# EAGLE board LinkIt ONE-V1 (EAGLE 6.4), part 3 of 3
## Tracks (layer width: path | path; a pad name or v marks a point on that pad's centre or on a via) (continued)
SMPSLDO_1V6  (via drill 0.3 pad 0.51) (continued)
  GND 0.406: C19.2 58.85,80.9 58.85,81.76 | 54.67,79.56 53.91,79.56 | 53.91,79.56 52.92,79.56 v52.91,79.58 | v54.28,80.77 54.28,79.96 | 54.28,79.96 54.28,79.93 53.91,79.56 | 54.28,79.96 54.67,79.56 | 58.85,81.76 58.85,82.35 v58.83,82.37 | v59.11,81.76 58.85,81.76 | v57.81,79.2 C19.2 | 54.67,79.56 57.47,79.56 | 57.47,79.56 57.52,79.56 C19.2 | 57.47,79.56 57.79,79.25
  Bottom 0.152: 58.29,81.51 U1.D10 58.28,81.55 58.45,81.71 59.05,81.71 v59.11,81.76 | U1.C3 U1.C2 54.23,81.02 54.23,80.77 v54.28,80.77 | U1.E10 58.5,82.05 v58.83,82.37
  Bottom 0.203: U1.A8 57.26,79.9 57.81,79.35 v57.81,79.2
  Bottom 0.305: 54.23,80.77 54.23,81.09 54.67,81.09 54.74,81.03
  Bottom 0.406: v52.91,79.58 51.54,79.58 C11.1 50.42,76.66 L6.1
SPI_MISO  (via drill 0.3 pad 0.51)
  Top 0.152: 26.95,103.86 v26.95,103.81 28.63,105.49 30.3,105.49 U11.13 | v34.57,90.02 34.57,89.59 34.93,89.23 37.47,89.23 38.18,88.52 41.07,88.52 42.09,89.53 46.71,89.53 47.73,88.52 51.49,88.52 52.55,87.45 60.91,87.45 61.87,86.49 U11.38
  Bottom 0.152: v26.95,103.81 26.99,103.77 U18.13 26.99,101.58 27.36,101.22 27.36,100.81 24.72,98.18 24.72,92.24 27.98,88.98 31.98,88.98 32.79,89.79 33.25,89.79 33.4,89.64 34.19,89.64 v34.57,90.02
SPI_MOSI  (via drill 0.3 pad 0.51)
  Top 0.152: U11.34 65.51,83.95 64.24,85.22 62.61,85.22 60.68,87.15 52.45,87.15 51.38,88.21 47.62,88.21 46.61,89.23 42.19,89.23 41.17,88.21 38.02,88.21 37.31,88.92 34.77,88.92 v33.58,90.12 | U11.12 32.54,105.18 28.98,105.18 v27.61,103.81
  Bottom 0.152: v27.61,103.81 27.61,102.49 27.66,102.44 27.66,102.25 U18.14 27.64,100.59 25.01,97.96 25.01,92.39 28.12,89.28 31.67,89.28 32.51,90.12 v33.58,90.12
SPI_SCL  (via drill 0.3 pad 0.51)
  Top 0.152: U11.37 63.37,83.95 60.48,86.84 52.35,86.84 51.28,87.91 47.52,87.91 46.51,88.92 42.29,88.92 41.28,87.91 37.82,87.91 37.11,88.62 34.47,88.62 33.71,89.38 33.07,89.38 v33,89.31 | U11.14 29.08,106.66 v26.24,103.81
  Bottom 0.152: v26.24,103.81 26.34,103.71 U18.12 | U18.12 | v33,89.31 32.36,88.67 27.86,88.67 24.4,92.14 24.4,98.36 26.29,100.25 26.29,100.46 26.29,102.17 U18.12
SPI_SS  (via drill 0.3 pad 0.51)
  Top 0.152: U11.11 35.94,106.81 34.01,104.88 29.34,104.88 v28.27,103.81
  Bottom 0.152: v28.27,103.81 U18.15
SQI_CE  (via drill 0.1 pad 0.25 layers 15-16, 0.2 pad 0.41 layers 2-15, 0.3 pad 0.51)
  GND 0.152: v36.26,79.43 36.92,79.43 37.24,79.75 37.24,80.16 36.91,80.49 36.91,86.69 v36.65,86.94
  GND1 0.076: v36.26,79.43 36.26,79.36 v36.07,79.16
  Bottom 0.102: 38.54,85.78 U3.1
  Bottom 0.152: v36.65,86.94 38.12,86.94 38.53,86.54 38.53,85.78 U3.1 | U7.G13 36.14,79.09 v36.07,79.16
SQI_SCK  (via drill 0.1 pad 0.25 layers 15-16)
  GND1 0.076: U7.G8 36.41,77 36.41,77.28 36.26,77.43 36.26,77.62 36.1,77.78 36.1,78.57 37.21,79.68 37.21,80.49 36.65,81.05 v36.65,81.15
  Bottom 0.102: U3.6 32.05,83.21 31.93,83.08 31.93,81.41 32.08,81.25 36.55,81.25 v36.65,81.15
  other vias: 36.14,76.73
SQI_SI  (via drill 0.1 pad 0.25 layers 15-16)
  GND1 0.076: v36.96,77.5 36.92,77.54 36.92,78.15 37.56,78.8 37.56,80.91 37.56,81.05 v37.16,81.46
  Bottom 0.076: U7.F9 36.59,77.13 v36.96,77.5
  Bottom 0.102: U3.5 32.81,81.6 32.95,81.46 v37.16,81.46
SQI_SIO2
  Bottom 0.076: U7.F12 36.54,78.43 36.54,78.45 36.54,79.43 36.86,79.75
  Bottom 0.102: 38.59,83.19 U3.3 38.59,83.24 39.35,83.24 39.6,82.98 39.6,81.66 39.59,81.66 39.29,81.36 38.46,81.36 36.86,79.75
SQI_SIO3  (via drill 0.1 pad 0.25 layers 15-16)
  GND1 0.076: v37.11,81.05 37.38,80.78 37.38,78.84 36.76,78.22 36.76,77.74 U7.F10
  Bottom 0.102: U3.7 31.95,84.48 31.67,84.2 31.67,81.3 31.93,81.05 36.3,81.05 36.55,80.8 36.86,80.8 v37.11,81.05
  other vias: 36.54,77.53
SQI_SO
  Bottom 0.076: 36.78,79.95 36.39,79.56 36.39,78.56 36.15,78.33 U7.G12
  Bottom 0.102: 38.54,84.51 U3.2 37.85,84.48 37.67,84.3 37.67,80.84 36.78,79.95
SW_SPI/SDIO  (via drill 0.3 pad 0.51)
  Top 0.152: U6.10 31.45,91.95 31.52,92.02 31.55,92.05 31.55,93.47 v31.52,93.5 | U6.2 26.59,92.45 v26.39,92.25 | v31.52,93.5 v31.52,93.49 v31.52,93.5 | SW1.COM 28.02,83.44 v27.46,84
  GND 0.152: v31.52,93.5 31.11,93.09 27.25,93.09 26.41,92.25 v26.39,92.25 25.02,90.88 v25.02,90.04
  Bottom 0.152: v25.02,90.04 26.92,88.14 26.92,86.61 27.56,85.98 27.56,84.1 v27.46,84
TR_N
  Bottom 0.114: L7.1 63.95,78.36 64.35,78.36 C141.1 64.59,78.54 64.77,78.36 65.05,78.36 arc45 65.22,78.43 65.53,78.74 65.86,78.74 U15.7
TR_P
  Bottom 0.076: 63.94,77.96 63.92,77.96 R61.1 | 64.85,77.95 64.83,77.95 C141.2
  Bottom 0.114: U15.5 65.56,77.51 65.19,77.88 arc45 65.01,77.95 64.85,77.95 | 63.94,77.96 64.35,77.96 C141.2
TRX_IO_N
  Bottom 0.114: U1.C10 58.3,81.05 58.31,81.04 arc45 58.52,80.96 58.58,80.96 arc-45 58.85,80.84 61.23,78.47 arc90 61.77,78.47 C142.1 61.9,78.56 62.1,78.36 62.55,78.36 L7.2
TRX_IO_P
  Bottom 0.114: U1.B10 58.3,80.55 arc-45 58.53,80.64 58.45,80.64 arc-45 58.72,80.53 61.14,78.11 arc45 61.41,78 61.46,78 arc-45 61.73,77.88 C142.2 62.13,77.94 62.13,77.96 62.58,77.96 62.58,77.94 R61.2
TX_EN  (via drill 0.1 pad 0.25 layers 1-2, 0.1 pad 0.25 layers 15-16, 0.2 pad 0.41 layers 2-15, 0.3 pad 0.51)
  Top 0.152: v45.44,80.24 45.44,74.78 46.97,73.25 46.97,66.85 50.55,63.27 v50.72,63.27
  GND 0.152: v45.44,80.24 44.83,80.24 44.02,81.05 v43.92,81.05
  GND1 0.102: v40.09,76.91 40.09,77.22 40.72,77.85 40.72,80.07 42.05,81.41 43.56,81.41 v43.92,81.05
  Bottom 0.076: U7.A9 38.54,77.15
  Bottom 0.102: U7.A9 39.88,77.13 v40.09,76.91
  Bottom 0.152: R55.2 R75.2 51.4,64.1 50.72,63.42 v50.72,63.27
TXO_HB
  Bottom 0.102: U7.C2 37.67,74.24 37.67,73.33
  Bottom 0.132: 37.67,73.33 37.67,70.43 arc45 37.78,70.16 40.9,67.04 arc45 41.17,66.93 48.32,66.93 arc45 48.7,67.08 49.01,67.4 arc-45 49.47,67.59 C134.1 L16.2
TXO_LB
  Bottom 0.102: U7.B2 38.14,74.31 37.93,74.09 arc45 37.87,73.97 37.87,73.62 arc45 37.93,73.47 37.97,73.43
  Bottom 0.132: 37.97,73.43 38.21,73.2 arc-45 38.33,72.91 38.33,70.7 arc45 38.44,70.43 41.24,67.63 arc45 41.51,67.52 47.94,67.52 arc45 48.14,67.6 49.24,68.69 arc-45 49.52,68.81 C135.1 L1.2
UART1_RX  (via drill 0.1 pad 0.25 layers 15-16, 0.2 pad 0.41 layers 2-15, 0.3 pad 0.51)
  Top 0.152: 30.87,102.44 R106.2 31.43,102.43 31.72,102.13 31.72,100.51 v31.77,100.46
  GND 0.152: v40.82,81.41 40.64,81.58 40.64,87.07 42.64,89.08 43.94,89.08 45.24,90.38 45.24,92.23 35.74,101.73 v35.74,101.85
  GND1 0.076: v37.18,77.18 37.34,77.18 37.44,77.28 38.08,77.28 38.15,77.21 38.61,77.21 38.93,77.53 39.33,77.53 39.98,78.19 39.98,78.79 39.63,79.14 39.63,80.06 39.74,80.18 39.74,81.04 40.11,81.41 v40.82,81.41
  Bottom 0.076: U7.E9 37.12,77.13 v37.18,77.18
  Bottom 0.152: v31.77,100.46 32.07,100.46 32.7,101.09 34.4,101.09 R82.2 35.34,101.85 v35.74,101.85 36.12,101.85 Q9.2 36.25,101.73
UART1_TX  (via drill 0.1 pad 0.25 layers 15-16, 0.2 pad 0.41 layers 2-15, 0.3 pad 0.51)
  Top 0.152: 27.5,102.43 26.8,101.73 v26.8,101.07
  Top 0.203: R107.2 27.5,102.43
  GND 0.152: v40.97,80.9 41.22,81.15 41.22,81.66 40.92,81.97 40.92,86.79 42.85,88.72 44.02,88.72 45.54,90.25 45.54,92.38 39.09,98.83 v39.09,99.75 | v26.8,101.07 30.5,101.07 33,98.58 35.18,98.58 v35.74,98.02
  GND1 0.076: U7.E8 37.13,76.73 37.53,77.12 38.01,77.12 38.09,77.05 38.8,77.05 38.96,76.89 39.24,76.89 40.34,77.98 40.34,79.5 39.9,79.93 39.9,80.7 40.11,80.9 v40.97,80.9
  GND1 0.102: 41.06,80.98 v40.97,80.9
  Bottom 0.152: v35.74,98.02 36.37,98.02 Q8.2 36.45,98.22 37.31,99.09 39.21,99.09 R46.2 39.46,99.38 v39.09,99.75
  other vias: 36.94,76.73
USB_5V  (via drill 0.3 pad 0.51, 0.38 pad 0.64)
  Top 0.152: R33.1 15.54,73.34 15.54,75.18 15.93,75.57 U12.2
  Top 0.406: 4.96,84.2 5.1,84.35 | U12.2 17.52,75.57 17.78,75.31 17.78,74.08 | 8,78.23 8,78.68 C49.+ | C106.1 17.82,73.7 v18.41,74.3
  Top 1.016: 5.1,84.35 5.18,84.35 v5.66,84.84
  GND 0.61: v7.75,77.34 5.84,77.34 3.05,74.55 3.05,65.53 v5.21,63.37 6.12,62.46 v6.12,58.74
  GND 2.032: 7.62,77.34 v7.75,77.34 8.64,77.34 9.91,77.34 10.03,77.34 10.67,76.71 11.05,76.33 13.08,74.3 v18.41,74.3
  Bottom 0.152: v18.41,74.3 18.41,74.4 18.92,74.91
  Bottom 0.203: R70.1 8.37,59.36 13.01,59.36 VCHG_5V1.T | 18.92,74.93 19.24,74.93 C74.1
  Bottom 0.406: 6.13,58.73 v6.12,58.74 | U8.4 4.83,58.74
  Bottom 0.61: 4.32,59.18 4.76,58.74 4.83,58.74 v6.12,58.74 C116.1 R70.1 | 4.19,63.25 Q14.2 v5.21,63.37 6.29,63.37 R93.1
  Bottom 1.778: v5.66,84.84 5.66,79.43 v7.75,77.34
  other vias: 18.03,74.93 19.05,74.17 6.98,77.34 7.37,77.98
  pour Top (isolate 0.254, no thermals): 3.63,84.81 5.26,84.81 5.26,83.85 3.63,83.85
  pour Bottom (isolate 0.254, no thermals): 17.53,75.56 17.53,74.3 arc90 17.78,74.04 19.56,74.04 arc90 19.81,74.3 19.81,75.56 arc90 19.56,75.82 17.78,75.82 arc90
  pour Top (isolate 0.254, no thermals): 17.53,74.42 17.4,74.42 arc90 17.14,74.17 17.14,73.71 arc90 17.4,73.46 19.05,73.46 arc90 19.3,73.71 19.3,75.18 arc90 19.05,75.44 17.78,75.44 17.78,74.68 arc-90
  pour Top (isolate 0.254, no thermals): 6.6,78.26 7.24,78.26 arc90 7.49,78.51 7.49,79.88 arc-90 7.75,80.14 8.64,80.14 arc-90 8.89,79.88 8.89,77.22 arc-90 8.64,76.96 6.6,76.96 arc-90 6.35,77.22 6.35,78 arc-90
USB_N
  Top 0.114: J7.2 5.53,83.33 5.71,83.14 6.59,83.14 | 6.59,83.14 7.56,83.14 R17.1 | 6.59,83.14 6.59,83.93 DP.T
USB_P
  Top 0.114: J7.3 5.57,82.68 5.71,82.82 6.6,82.82 | 6.6,82.82 7.69,82.82 R18.1 | 6.6,82.82 DN.T
USBD_N  (via drill 0.3 pad 0.51)
  Top 0.114: R17.2 9.02,83.64 9.47,83.19 10.09,83.19 10.24,83.34 D6.1 12.81,83.92 13.54,83.19 21.27,83.19 25.95,78.52 31.84,78.52 32.23,78.13 v32.23,77.9
  Bottom 0.076: U7.N11 33.49,77.68 32.46,77.68 v32.23,77.9
  Bottom 0.102: U7.N11 33.7,77.93
USBD_P  (via drill 0.3 pad 0.51)
  Top 0.114: R18.2 9.05,82.45 9.47,82.87 10.09,82.87 10.24,82.73 D6.2 12.81,82.14 13.54,82.87 21.14,82.87 25.82,78.2 31.52,78.2 v31.62,78.1
  Bottom 0.076: U7.P11 32.92,77.93 32.51,78.34 31.86,78.34 v31.62,78.1
VA  (via drill 0.1 pad 0.25 layers 1-2, 0.1 pad 0.25 layers 15-16, 0.2 pad 0.41 layers 2-15)
  Top 0.152: v31.93,74.3 32.12,74.3 C94.1
  GND 0.132: v32.33,74.3 v31.93,74.3 v32.33,74.3
  GND1 0.132: v32.74,74.4 32.64,74.3 v32.33,74.3
  Bottom 0.152: 33.33,74.73 U7.P3 33.27,74.73 32.94,74.4 v32.74,74.4
VBAT  (via drill 0.1 pad 0.25 layers 1-2, 0.1 pad 0.25 layers 15-16, 0.2 pad 0.41 layers 2-15, 0.3 pad 0.51)
  Top 0.152: 37.3,73.1 37.14,73.1 v36.78,73.46 | 41.1,65.58 41.1,65.63 v41.17,65.71
  Top 0.203: 34.8,76.36 C72.1 | 36.07,62.36 37.52,62.36 v37.67,62.2 | v34.72,74.7 34.72,74.77 C101.1
  Top 0.254: U20.6 21.9,67.11 21.34,66.55 19.56,66.55 18.99,67.11 U20.3
  Top 0.305: C33.+ 40.44,62.74 40.46,62.76 40.46,62.92 | 37.33,73.18 C8.1 | R78.2 12.76,58.86 13.46,59.56 15.88,59.56 v16.13,59.31
  Top 0.406: v33.96,76.38 C72.1 | C3.1 30.73,66.8 30.17,66.24
  Top 0.61: U4.1 52.77,91.12 C45.1 52.4,91.06 v51.41,90.07 | 37.59,71.88 C73.1 | C73.1 37.35,72.12 C8.1 37.3,73.1 37.28,73.1 35.33,75.06 35.07,75.06 C101.1 35.03,75.82 34.81,76.03 C72.1 34.82,76.36 | 38.25,66.02 38.25,65.81 37.85,65.41 | 38.25,66.02 38.25,66.06 | 38.25,66.06 38.25,71.22 C73.1 | v51.13,66.67 50.42,67.39 50.42,77.52 | 50.42,77.52 50.42,77.6 48.64,79.38 48.64,81.47 v48.88,81.71 | 50.42,77.52 L2.1 | 38.25,66.02 38.86,65.41 | 38.25,66.06 37.72,65.53
  Top 1.016: C50.+ 30.8,65.62 30.79,65.63 | v41.17,65.71 40.87,65.41 38.86,65.41 37.85,65.41 v36.65,65.41 v35.89,65.41
  Top 1.27: v35.89,65.41 35.64,65.41 v35.13,65.91
  Top 2.032: C30.+ C33.+ | 35.94,62.48 36.07,62.36 36.07,62.51 C30.+ | C30.+ 35.89,62.69 v35.89,65.41 35.71,65.58 30.84,65.58 30.79,65.63 30.17,66.24 28.3,68.12 27.06,68.12 L8.1
  GND 0.152: v60.43,63.93 60.43,64.59 61.09,64.59 v61.14,64.64 60.45,64.64 | 60.43,65.15 v60.38,65.2 | v37.67,62.2 37.67,62.31 v38.18,62.81 38.23,62.76 38.23,62.74 | v38.63,62.23 38.63,62.33 38.23,62.74 | 38.23,62.74 38.23,62.36 | v34.27,74.45 34.47,74.45 v34.72,74.7 | v33.93,70.08 33.48,69.62 33.15,69.62 32.74,70.03 29.29,70.03 28.42,70.89 13.39,70.89 11.1,73.18 6.43,73.18 6.22,72.97 SW3.COM2 | v36.6,73.74 36.6,73.63 v36.78,73.46
  GND 0.203: v33.96,76.38 33.96,76.76 33.81,76.91 v33.81,77.57
  GND 0.305: 17.53,69.22 17.53,69.62 | v15.24,68.77 15.24,69.49 | 15.24,69.49 15.37,69.62 | 15.24,69.49 15.24,69.8 15.27,69.83
  GND 0.61: v41.17,65.71 50.16,65.71 v51.13,66.67 | v51.41,90.07 50.01,88.67 50.01,82.84 v48.88,81.71
  GND 2.032: 60.45,64.64 57.79,64.64 54.17,61.02 39.56,61.02 38.23,62.36 | SW3.COM1 SW3.COM2 10.57,71.88 12.83,69.62 15.37,69.62 17.53,69.62 27.84,69.62 32.05,65.41 v35.89,65.41
  GND1 0.102: U7.M10
  GND1 0.132: U7.E1 36.75,73.74 v36.6,73.74
  GND1 0.152: U7.L3 v34.27,74.45 | v33.81,77.57 34.1,77.57 U7.M10
  Bottom 0.102: U7.H1 35.74,73.89 35.64,73.79 35.64,73.18 34.21,71.75 34.21,71.14 33.93,70.87 v33.93,70.08
  Bottom 0.152: C128.2 60.38,64.64 | 60.38,64.64 60.43,64.59 | 60.38,64.64 v61.14,64.64
  Bottom 0.305: U14.26 56.56,65.26 56.77,65.05 | v16.13,59.31 15.68,59.76 15.68,63.88 | 15.68,63.88 15.68,66.23 15.88,66.42 15.88,66.41 D2.2 15.89,68.12 15.83,68.18 v15.24,68.77 | 15.68,63.88 15.43,63.63 VBAT_TP.T 15.37,63.63 15.62,63.37
  other vias: 34.54,74.73 34.14,77.53 36.94,73.93
  pour Bottom (isolate 0.254, no thermals): 56.46,66.42 56.67,66.42 56.67,65.76 56.93,65.51 60.86,65.51 arc-90 61.49,64.87 61.49,64.36 arc-90 60.86,63.73 58.62,63.73 arc-90 58.24,64.11 arc90 57.61,64.74 56.46,64.74
  pour Top (isolate 0.254, no thermals): 22.22,67.31 23.57,67.31 23.75,67.49 23.75,68.83 arc-90 24.38,69.47 28.45,69.47 arc-90 29.08,68.83 29.08,67.49 arc-90 28.45,66.98 22.22,66.98
VCDT  (via drill 0.1 pad 0.25 layers 15-16, 0.3 pad 0.51)
  GND 0.152: v31.22,69.42 31.22,68.61 32.33,67.49 v32.33,67.13 | v8.28,57.84 8.28,61.48 9.16,62.36 9.91,62.36 10.41,61.85 16.76,61.85 v17.27,62.36
  GND1 0.102: v35.33,75.13 35.33,73.83 34.12,72.62 33.35,72.62 33.2,72.47 33.2,72.11 v33.15,72.06
  Bottom 0.102: 35.35,75.13 U7.J4 v35.33,75.13
  Bottom 0.152: v33.15,72.06 33.15,71.68 31.22,69.75 v31.22,69.42 | v32.33,67.13 23.24,67.13 18.72,62.61 17.53,62.61 v17.27,62.36 | R86.1 8.78,57.84 v8.28,57.84 7.76,57.84 R70.2
VCORE  (via drill 0.1 pad 0.25 layers 15-16, 0.3 pad 0.51)
  Top 0.406: 38.23,78.1 38.28,78.16 | 38.23,78.1 38.28,78.1 | 38.28,78.1 37.67,77.5 33.26,77.5 v32.88,77.12 | 38.28,78.1 39.02,78.1 v39.07,78.05 | 38.23,78.1 38.23,78.12 C69.1
  GND1 0.076: v32.88,77.12 U7.P9
  Bottom 0.152: U7.A11 38.94,77.93 v39.07,78.05
  other vias: 33.34,77.13
VIO18_LDO  (via drill 0.3 pad 0.51)
  Top 0.406: v32.94,79.78 33.15,79.78 33.41,80.05 R37.1 C70.1 32.27,80.91 31.77,81.41 30.96,81.41 v30.61,81.05
  Bottom 0.152: U7.P13 U7.N13 33.74,79.19 33.15,79.78 v32.94,79.78
  Bottom 0.406: 30.77,86.31 31.56,87.1 34.87,87.1 35.94,88.16 39.35,88.16 39.84,87.66 40.59,87.66 41.09,88.16 R114.1 | 30.77,86.31 30.71,86.24 | 30.77,86.31 30.77,86.3 30.56,86.08 30.56,81.1 v30.61,81.05 | 41.68,89.53 41.5,89.71 41.5,89.76 Q11.1 | 41.07,93.13 R118.1 41.58,93.14 | 41.78,92.96 41.78,90.04 Q11.1 | 41.78,92.96 41.78,93.34 | 41.78,93.34 41.78,94.28 Q13.1 41.55,94.51 42.17,95.13 42.17,99.21 41.99,99.39 41.54,99.39 R115.1 41.5,101.5 Q12.1 | 41.58,93.14 41.78,93.34 | 41.58,93.14 41.61,93.14 41.78,92.96 | Q11.1 41.09,89.34 R114.1 | 41.15,88.38 41.11,88.38 R114.1
VIO28_LDO  (via drill 0.3 pad 0.51)
  Top 0.152: v52.91,83.21 52.98,83.21 54.08,84.3 54.97,84.3 55.27,84.61 56.17,84.61 C23.1
  Top 0.203: R53.2 v6.98,107.06 | v39.29,76.35 40.14,76.35 40.16,76.38
  Top 0.406: C71.1 C63.1 38.34,76.35 v39.29,76.35 40,76.35 R67.1 40.16,76.38 40.77,76.38 41.22,76.83 42.55,76.83 | C23.1 56.74,85.2 v56.74,86.23 56.74,86.34 arc-45 56.77,86.4 | 58.19,86.4 60.12,86.4 60.59,85.92 R92.2 R87.2 | v58.45,85.52 58.45,86.13 | v42.55,87.71 42.7,87.86 46.17,87.86 47.19,86.84 51.61,86.84 52.06,86.4 56.77,86.4 | v45.97,81.74 45.87,81.74 44.76,80.62 44.21,80.62 42.8,79.21 42.8,77.09 | 42.8,76.58 42.8,73.86 43.21,73.46 v43.21,63.09 43.21,60.88 44.27,59.82 46.97,59.82 47.62,59.16 v47.62,58.8 | 42.8,76.58 42.8,77.09 | 42.55,76.83 42.8,77.09 | 42.55,76.83 42.8,76.58 | 56.77,86.4 58.19,86.4 | 58.19,86.4 58.45,86.14 58.45,86.13 | 58.45,86.13 58.65,86.33 | R76.2 29.16,102.56 28.52,103.2 26.39,103.2 | 26.39,103.2 25.98,103.2 | 26.19,103 25.98,103.2 | R77.2 26.19,103 | 26.19,103 26.39,103.2 | 19.84,103.2 v19.79,103.15 20.27,103.63 22.45,103.63 | v42.95,95.83 41.02,95.83 39.29,97.56 v38.23,97.56 | v38.12,92.63 41.71,92.63 v42.52,93.45 | 25.98,103.2 25.96,103.2 25.53,103.63 22.99,103.63 | 22.99,103.63 22.45,103.63 | R49.2 22.73,103.35 | 22.73,103.35 22.73,103.38 22.99,103.63 | 22.73,103.35 22.45,103.63
  Top 0.61: C14.2 54.83,80.3 v55.27,80.75
  GND 0.305: v30.86,95.07 | v30.86,95.07 28.99,95.07 26.8,97.26 23.44,97.26 21.31,95.12 v20.5,95.12 19.79,95.83 v19.79,103.15 | v6.98,107.06 7.34,107.06 10.03,104.37 18.57,104.37 v19.79,103.15 | 19.79,102.74 v19.79,103.15 | v30.86,95.07
  GND 0.406: 55.25,80.7 55.27,80.72 v55.27,80.75 55.9,80.12 57.21,80.12 58.15,81.06 58.15,84.51 58.45,84.81 v58.45,85.52 | v47.62,58.8 47.62,57.53 46.97,56.87 25.07,56.87 22.11,59.83 22.05,59.89 v22.05,60.76 | v33.1,92.43 33.15,92.43 33.25,92.53 33.25,93.43 32.04,94.64 31.29,94.64 v30.86,95.07
  Bottom 0.102: U7.B7 38.14,76.34 38.12,76.33
  Bottom 0.152: U1.H1 53.48,83.55 53.15,83.21 v52.91,83.21 | U1.D3 55.27,81.03 v55.27,80.75 | U17.6 45.66,62.49 45.44,62.71 45.44,63.47 45.14,63.78 44.56,63.78 U17.3 | 21.25,60.5 R36.2 | VIO_28.T 16.73,63.08 16.73,61.63 17.14,61.21 19.54,61.21 R81.2
  Bottom 0.203: U1.J7 U1.K7 56.76,86.22 v56.74,86.23 | 38.12,76.33 38.12,76.71 U7.B8 | 38.14,76.34 39.28,76.34 v39.29,76.35
  Bottom 0.254: v58.45,85.52 58.45,84.91 58.26,84.72 U1.K10
  Bottom 0.305: U17.3 43.07,63.79 C122.1 42.98,63.7 | 20.26,60.5 R81.2 R36.2 21.81,60.52 v22.05,60.76
  Bottom 0.406: R69.1 C5.1 32.32,98.36 30.88,96.91 U18.2 30.88,95.08 v30.86,95.07 | Q3.1 31.48,92.48 R98.1 32.22,92.43 v33.1,92.43 33.86,92.43 34.9,91.39 Q4.1 36.34,91.39 R99.1 | C122.1 43.21,63.52 v43.21,63.09 | v45.97,81.74 45.97,83.19 42.55,86.61 v42.55,87.71 42.55,93.42 v42.52,93.45 42.52,94.18 42.95,94.61 v42.95,95.83 | v20.5,95.12 20.43,95.19 20.02,95.19 R38.1 | 36.39,91.44 R99.1 | 37.34,93.08 37.34,93.65 Q10.1 | 37.34,92.46 37.95,92.46 v38.12,92.63 | 37.34,92.46 36.77,92.46 36.51,92.19 R99.1 | R82.1 35.27,102.84 35.43,102.84 35.74,102.54 37.21,102.54 Q9.1 38.23,101.27 39.09,100.41 39.8,100.41 40.16,100.05 40.16,98.96 39.69,98.49 R46.1 38.6,98.49 38.08,97.97 38.1,97.97 Q8.1 v38.23,97.56 | 37.34,92.46 37.34,93.08 | 37.34,93.08 R112.1
VIO33_LDO  (via drill 0.3 pad 0.51)
  Top 0.305: U6.14 29.59,94.78 C87.1
  Top 0.406: 31.5,94.41 31.5,98.88 31.19,99.19 30.32,99.19 29.98,99.53 29.98,103 30.4,103.43 v30.86,103.43 30.86,103.4 | v35.08,94.06 35.08,94.11 34.22,93.25 32.65,93.25 31.5,94.41 | 31.5,94.41 30.86,94.41 | 30.86,94.41 30.61,94.41 30.05,94.97 C87.1 | v30.86,94.03 30.86,94.41
  GND 0.406: v41.94,102.79 41.89,102.79 40.21,104.47 31.32,104.47 30.86,104.01 v30.86,103.43 | v29.74,85.57 29.74,88.47 30.61,89.33 30.61,90.75 32.59,92.74 32.59,93.29 31.78,94.1 30.93,94.1 | 30.93,94.1 v30.86,94.03 30.93,94.1
  GND 0.61: v11.46,88.92 13.71,86.67 19.03,86.67 19.99,87.63 19.99,89.53 24.11,93.65 30.48,93.65 v30.86,94.03 | v31.37,63.88 31.24,63.88 27.05,68.07 12.07,68.07 v10.92,69.22
  Bottom 0.152: 31.95,94.28 32.02,94.28 R73.2 | R83.2 35.26,98.6
  Bottom 0.203: 30.86,102.24 U18.19
  Bottom 0.406: v30.86,103.43 30.88,103.41 U18.19 30.88,101.34 31.11,101.1 32.1,101.1 C7.1 34.04,102.02 R111.2 | 35.26,98.6 35.05,98.6 34.32,97.87 34.32,95.38 34.63,95.06 R113.2 35.1,94.08 v35.08,94.06 | R117.2 R119.2 44.86,102.09 R116.2 42.61,102.12 v41.94,102.79 | R20.1 29.55,85.33 29.74,85.52 v29.74,85.57 | v30.86,94.03 30.04,94.03 R71.2 | v30.86,94.03 30.86,94.06 | 32.04,94.21 R73.2 31.97,94.13 31.01,94.13 30.91,94.03 v30.86,94.03
  Bottom 0.61: v11.46,88.92 11.46,87.1 10.25,85.89 10.25,85 11.81,83.44 11.81,70.1 v10.92,69.22 | R116.2 45.11,101.89 C2.1 45.11,98.53 C32.1 45.14,96.44 U19.4 | v31.37,63.88 31.37,59.31 U11.31 30.61,58.42 32.13,56.9 34.04,56.9 U11.29
  pour Bottom (isolate 0.254, no thermals): 47.73,97.41 44.32,97.41 arc90 43.69,96.65 43.69,94.41 arc90 44.32,93.78 47.73,93.78 arc90 48.36,94.41 48.36,96.65 arc90
VMC  (via drill 0.1 pad 0.25 layers 15-16, 0.3 pad 0.51)
  Top 0.305: v24.75,77.99 25.96,76.78 30.64,76.78 31.2,76.22 C95.1 31.2,76.16 31.65,76.61 31.65,76.76 v31.67,76.78
  GND1 0.076: 32.81,76.73 32.95,76.73 33.36,76.33 33.55,76.33 33.98,76.76 34.57,76.76 U7.K9
  GND1 0.102: v31.67,76.78 31.78,76.67 32.58,76.67 32.64,76.73 32.81,76.73
  Bottom 0.305: 19.16,86.75 19.21,86.8 J4.4 19.85,86.8 20.55,87.5 R72.1
  Bottom 0.406: R2.1 R74.1 22.17,83.48 22.17,82.93 21.78,82.54 21.78,81.39 | 19.16,86.75 18.47,86.05 18.47,81.48 18.82,81.13 21.49,81.13 | 21.49,81.13 21.51,81.13 21.78,81.39 | v24.75,77.99 23.96,77.99 21.78,80.17 21.78,81.39 | 21.49,81.13 21.72,80.9 | C66.1 21.46,86.63 21.46,87.49 R72.1
  other vias: 34.94,77.13
VREF
  Bottom 0.152: U7.G1 36.14,73.31 34.7,71.87 C92.1
VRTC  (via drill 0.1 pad 0.25 layers 1-2, 0.1 pad 0.25 layers 15-16, 0.2 pad 0.41 layers 2-15)
  Top 0.406: D1.+ 18.29,86.54 18.29,85.34 19.3,84.33 21.46,84.33 | 21.84,84.33 21.46,84.33 | R8.1 21.65,84.52 | 21.65,84.52 21.46,84.33 | 21.65,84.52 21.84,84.33 | v30.4,79.58 30.35,79.63 26.92,79.63 26.54,80.01 26.54,80.97 25.97,81.53 24.89,81.53 22.1,84.33 21.84,84.33
  GND 0.203: v30.4,79.58 31.32,79.58 32.79,78.1 32.79,77.75 32.36,77.32 v32.3,77.32
  GND1 0.102: v32.3,76.99 v32.3,77.32
  Bottom 0.102: U7.P8 32.56,76.73 v32.3,76.99
VSF  (via drill 0.1 pad 0.25 layers 1-2, 0.1 pad 0.25 layers 15-16, 0.2 pad 0.41 layers 2-15, 0.3 pad 0.51)
  Top 0.152: v36.84,78.14 36.83,78.13
  Top 0.406: C47.1 v36.84,78.14
  GND 0.406: v36.2,87.5 36.25,87.55 36.96,87.55 37.31,87.2 37.31,80.7 37.64,80.37 37.64,79.61 v36.95,78.92 36.84,78.82 v36.84,78.14
  GND1 0.305: v36.38,78.02 36.38,78.35 v36.95,78.92
  Bottom 0.076: U7.F11 36.48,77.93 v36.38,78.02
  Bottom 0.406: U3.8 31.42,85.75 | 31.42,85.75 31.25,85.75 C91.1 | v36.2,87.5 35.21,86.52 31.81,86.52 31.42,86.13 31.42,85.75
VSIM1  (via drill 0.1 pad 0.25 layers 1-2, 0.1 pad 0.25 layers 15-16, 0.2 pad 0.41 layers 2-15, 0.3 pad 0.51)
  Top 0.152: v32.64,75.21 32.39,74.95 | C97.1 31.2,74.74
  Top 0.305: v30.96,74.93 31.01,74.93 31.2,74.74 32.17,74.74 v32.64,75.21
  GND 0.102: v33,75.41 32.79,75.21 v32.64,75.21
  GND 0.152: v5.1,94.28 5.1,94.26 5.77,93.6 8.76,93.6 v8.92,93.75 9.27,93.4 9.27,88.11 12.83,84.56 23.39,84.56 24.51,83.44 27.36,83.44 27.96,82.83 27.96,77.44 30.45,74.95 30.96,74.95 v30.96,74.93
  GND1 0.076: U7.L7 34.54,75.94 34.21,75.62 33.2,75.62 v33,75.41
  GND1 0.102: U7.L7 34.54,76.41
  Bottom 0.152: J4.C1 5.13,97.04 C65.1
  Bottom 0.203: J4.C1 5.13,94.31 v5.1,94.28 | J4.C6 8.94,93.77 v8.92,93.75
  other vias: 34.54,76.33
VSIM2  (via drill 0.3 pad 0.51)
  Top 0.152: C9.1 v36.2,79.98
  Bottom 0.076: v36.2,79.98 35.94,79.73 35.94,79.48 35.74,79.28 U7.H13
VUSB  (via drill 0.3 pad 0.51)
  Top 0.152: C10.1 32.27,79.41 32.54,79.15 32.92,79.15 v32.94,79.12
  Bottom 0.076: U7.P12 33.23,78.33
  Bottom 0.152: v32.94,79.12 32.94,78.61 33.23,78.33
WIFI_BT_PRI  (via drill 0.1 pad 0.25 layers 1-2, 0.1 pad 0.25 layers 15-16, 0.2 pad 0.41 layers 2-15, 0.3 pad 0.51)
  Top 0.152: R5.1 56.22,84.3 55.45,84.3 55.13,83.98 54.34,83.98 52.07,81.71 50.65,81.71 50.14,82.22 45.75,82.22 44.58,81.05 41.68,81.05 40.73,80.1 39.89,80.1 v39.8,80.19
  Top 0.406: R5.1 56.78,83.58 v57.28,83.08
  GND 0.152: v20.32,99.16 20.42,99.06 21.97,99.06 22.15,98.88 31.42,98.88 32.64,97.66 34.37,97.66 37.92,94.11 38.23,94.11 40.11,92.23 40.11,83.24 40.36,82.98 40.36,81.25 39.8,80.7 v39.8,80.19 39.55,80.19 38.73,79.38 v38.53,79.38
  GND1 0.102: v38.02,79.38 v38.53,79.38
  Bottom 0.076: U1.H7 | 37.75,78.33 U7.C12 37.74,79.09 v38.02,79.38
  Bottom 0.152: U1.H7 57.23,83.08 v57.28,83.08 | v20.32,99.16 20.32,99.53 R68.2
WIFI_EN  (via drill 0.1 pad 0.25 layers 15-16, 0.2 pad 0.41 layers 2-15, 0.3 pad 0.51)
  GND 0.102: v40.62,75.01 40.72,75.01 41.68,75.97 41.68,76.73 42.29,77.34 42.44,77.34
  GND 0.152: 42.44,77.34 50.55,77.34 51.56,78.36 54.67,78.36 v55.23,78.92
  GND1 0.076: U7.C3 38.18,75.16 38.76,75.16 39.17,74.75 39.47,74.75 39.77,74.46 40.07,74.46 v40.62,75.01
  Bottom 0.076: U1.B5 55.5,80.29 55.5,79.48
  Bottom 0.152: 55.5,79.48 55.5,79.18 v55.23,78.92
  Bottom 0.203: R3.1 55.23,77.79 v55.23,78.92
  other vias: 37.74,74.73
WIFI_MC1CLK  (via drill 0.1 pad 0.25 layers 1-2, 0.1 pad 0.25 layers 15-16, 0.2 pad 0.41 layers 2-15, 0.3 pad 0.51)
  Top 0.152: v51.71,83.08 51.66,83.13 40.46,83.13 39.14,81.81 v35.38,81.81
  GND 0.152: v35.38,81.3 v35.38,81.81
  GND1 0.152: v35.38,81.3 35.38,80.72 35.18,80.52 v35.18,80.44
  Bottom 0.076: v35.18,80.44 35.38,80.24 35.38,79.68 35.19,79.49 35.19,78.57 U7.K12 | U1.J2 54.26,84.07 54.03,84.3 53.57,84.3 53.32,84.56
  Bottom 0.152: 53.32,84.56 53.22,84.65 52.25,84.65 51.84,84.24 51.84,83.21 v51.71,83.08
WIFI_MC1CMD  (via drill 0.1 pad 0.25 layers 1-2, 0.1 pad 0.25 layers 15-16, 0.2 pad 0.41 layers 2-15, 0.3 pad 0.51)
  Top 0.152: v34.37,81.81 35.08,82.53 38.73,82.53 39.95,83.74 50.98,83.74 51.23,84 51.94,84 52.3,83.64 52.71,83.64 v53.16,84.1
  GND 0.076: v34.37,81.3 v34.37,81.81
  GND1 0.152: v34.27,80.49 34.27,81.2 v34.37,81.3
  Bottom 0.076: U7.L13 34.54,79.5 34.27,79.78 v34.27,80.49
  Bottom 0.152: v53.16,84.1 53.7,84.1 U1.J1
WIFI_MC1DA0  (via drill 0.1 pad 0.25 layers 1-2, 0.1 pad 0.25 layers 15-16, 0.2 pad 0.41 layers 2-15, 0.3 pad 0.51)
  Top 0.152: v52.35,82.88 52.35,83.13 51.92,83.57 51.31,83.57 51.18,83.44 40.21,83.44 38.99,82.22 35.28,82.22 v34.87,81.81
  GND 0.076: v34.87,81.3 v34.87,81.81
  GND1 0.152: v34.67,80.49 34.67,81.1 v34.87,81.3
  Bottom 0.076: 34.94,78.8 U7.K13 34.94,79.33 34.52,79.76 34.52,80.34 v34.67,80.49 | U1.H3 54.76,83.51 54.53,83.29 53.62,83.29 53.42,83.08 53.42,82.98
  Bottom 0.152: 53.42,82.98 53.42,82.93 53.24,82.75 52.48,82.75 v52.35,82.88
WIFI_MC1DA1  (via drill 0.1 pad 0.25 layers 1-2, 0.1 pad 0.25 layers 15-16, 0.2 pad 0.41 layers 2-15, 0.3 pad 0.51)
  Top 0.152: v33.35,81.81 34.67,83.13 38.28,83.13 39.5,84.35 50.57,84.35 50.93,84.71 53.34,84.71 54.48,84.71 v54.79,85.01
  GND 0.152: v33.35,81.81 v33.35,81.3
  GND1 0.152: v33.35,80.49 v33.35,81.3
  Bottom 0.076: v33.35,80.49 33.35,80.22 34.14,79.43 U7.M12
  Bottom 0.152: v54.79,85.01 54.79,84.08 U1.J3
WIFI_MC1DA2  (via drill 0.1 pad 0.25 layers 1-2, 0.1 pad 0.25 layers 15-16, 0.2 pad 0.41 layers 2-15, 0.3 pad 0.51)
  Top 0.152: v33.86,81.81 34.87,82.83 38.53,82.83 39.75,84.05 50.78,84.05 51.05,84.33 52.32,84.33 v52.5,84.15
  GND 0.076: v33.86,81.3 v33.86,81.81
  GND1 0.152: v33.86,80.49 v33.86,81.3
  Bottom 0.076: v33.86,80.49 33.86,79.94 34.29,79.52 34.29,78.58 U7.L12 | U1.H2 54.26,83.56 54.03,83.8 53.42,83.8 53.26,83.64 53.01,83.64 v52.5,84.15
WIFI_MC1DA3  (via drill 0.1 pad 0.25 layers 1-2, 0.1 pad 0.25 layers 15-16, 0.2 pad 0.41 layers 2-15, 0.3 pad 0.51)
  Top 0.152: v54.23,85.42 53.82,85.01 50.8,85.01 50.44,84.66 39.24,84.66 38.02,83.44 34.47,83.44 v32.84,81.81
  GND 0.076: v32.84,81.3 v32.84,81.81
  GND1 0.152: v32.84,80.49 v32.84,81.3
  Bottom 0.076: 33.74,78.34 U7.N12 33.74,78.35 33.98,78.59 33.98,79.35 v32.85,80.49 v32.84,80.49
  Bottom 0.152: v54.23,85.42 54.23,84.57 U1.K2
WIFI_OSC_EN  (via drill 0.1 pad 0.25 layers 15-16, 0.2 pad 0.41 layers 2-15, 0.3 pad 0.51)
  GND 0.102: 42.44,77.04 42.31,77.04 41.86,76.59 41.86,75.89 41.02,75.06 41.02,74.91 40.62,74.5 v40.56,74.5
  GND 0.152: 42.44,77.04 50.67,77.04 51.69,78.05 58.75,78.05 59.61,78.92 59.61,82.4 v58.98,83.03
  GND1 0.076: 38.14,74.77 38.38,75.01 38.66,75.01 39.09,74.57 39.4,74.57 39.69,74.28 40.11,74.28 40.34,74.5 v40.56,74.5
  GND1 0.102: U7.B3 38.14,74.77
  Bottom 0.076: U1.F9 57.88,82.55 58.13,82.8 58.39,82.8 58.4,82.8
  Bottom 0.152: v58.98,83.03 58.75,83.03 58.52,82.8 58.4,82.8
  other vias: 38.14,74.73
WIFI_RST_N  (via drill 0.1 pad 0.25 layers 15-16, 0.2 pad 0.41 layers 2-15, 0.3 pad 0.51)
  GND 0.102: 42.49,77.65 42.29,77.65 41.5,76.86 41.5,76.06 40.78,75.34 40.44,75.34 39.9,74.8 v39.9,74.78
  GND 0.152: v57.86,85.06 57.73,84.94 57.73,82.88 55.92,81.06 55.67,81.06 55.45,81.28 53.93,81.28 50.3,77.65 42.49,77.65
  GND1 0.076: U7.C4 37.92,75.31 38.84,75.31 39.21,74.94 39.74,74.94 v39.9,74.78
  GND1 0.102: U7.C4
  Bottom 0.152: U1.K9 57.76,84.96 v57.86,85.06
  other vias: 37.74,75.13
WIFI_RTC  (via drill 0.1 pad 0.25 layers 15-16, 0.2 pad 0.41 layers 2-15, 0.3 pad 0.51)
  Top 0.152: v45.41,87.25 45.36,87.2 45.01,87.2 44.6,86.79 37.77,86.79 36.96,85.98 35.18,85.98 31.37,89.79 v31.37,89.84
  GND 0.152: v45.41,87.25 45.41,87.07 42.9,84.56 42.9,80.9 42.29,80.29 v42.29,80.09 42.29,80.03 43.05,79.27 47.99,79.27 49.7,80.99 v50,80.99 | v31.37,89.84 31.32,89.84 33.66,92.18 33.66,93.61 32.22,95.05 31.64,95.05 31.15,95.53 29.08,95.53 26.95,97.66 22.78,97.66 v22.63,97.51
  GND1 0.076: 40.31,76.63 40.21,76.53 40.21,76.17 40.02,75.98 37.29,75.98 U7.E7
  GND1 0.102: 40.31,76.63 40.72,77.04 40.72,77.14 41.12,77.55 41.12,79.78 41.43,80.09 v42.29,80.09
  Bottom 0.152: R39.1 22.63,99.22 v22.63,97.51 | 49.78,81.28 49.8,81.28 R32.2 49.82,81.17 v50,80.99
  other vias: 36.94,76.33
WIFI_XIN
  Bottom 0.152: U1.D1 50.95,81.55 R32.1
XIN  (via drill 0.1 pad 0.25 layers 15-16)
  GND1 0.076: U7.M7 34.11,76.33 33.76,75.97 32.59,75.97 v32.54,76.02
  Bottom 0.152: v32.54,76.02 31.52,76.02 30.86,76.68 30.86,78.1 30.5,78.46 30.2,78.46 29.64,79.02 | 29.64,79.02 29.58,79.02 X1.1 | C75.1 29.83,79.21 29.64,79.02
  other vias: 34.14,76.33
XMIC  (via drill 0.3 pad 0.51)
  Top 0.305: L21.1 17.27,99.95 17.27,98.98 D3.2 17.35,96.54 17.04,96.24 17.04,94.72 16.74,94.41 16.74,92.81 v16.64,92.71
  Bottom 0.152: R14.1 27.06,76.33
  Bottom 0.305: v16.64,92.71 17.35,92.71 18.11,91.95 18.11,87.53 16.94,86.36 16.94,80.87 18.18,79.63 20.57,79.63 23.75,76.45 26.94,76.45 27.06,76.33 27.06,75.57 arc-45 26.95,75.3 26.9,75.25 | 26.9,75.25 C59.1 R13.1 28.96,75.25 C58.2 | 26.9,75.25 26.11,75.25 C56.1 | 27.05,76.44 R14.1
XMP3_L
  Top 0.203: D3.1 19.13,100.33
  Top 0.305: 19.13,100.33 L22.1 | D3.1 19.13,95.87 R16.1 C54.1 R10.2
XMP3_R
  Top 0.305: L23.1 16,99.21 D4.1 16,95.85 R15.1 C53.1 R11.2
XOUT  (via drill 0.1 pad 0.25 layers 15-16)
  GND1 0.076: U7.M6 34.14,75.9 34.06,75.82 32.74,75.82 v32.54,75.62
  Bottom 0.152: v32.54,75.62 32.44,75.72 31.37,75.72 30.56,76.53 30.56,77.95 30.35,78.16 30.1,78.16 29.64,77.7 29.63,77.7 X1.2 29.91,77.19 C76.1
  other vias: 34.14,75.93

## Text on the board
tPlace: NC | D9 | D8 | D7 | D6 | D5 | D4 | D3 | D2 | D1 | D0 | SCL | SDA | GND | D13 | D12 | D11 | D10 | ~ | ~ | TX | RX | RX | SCL | TX | SDA | 5V | 5V | GND | GND | SPI | - | + | - | + | SD | MISO | NC | SCK | MOSI | MS | USB | NC | GND | PWR_SW | UART | BAT | LinkIt ONE | v1.0 08/08/2014 | by Seeed Studio | www.seeedstudio.com | + | RST | NC | IOR | RST | 3V3 | 5V | GND | GND | NC | A0 | A1 | A2 | NC | SDA | SCL | -
bPlace: RESET | RST_B | TRTCK | TDI | GND | TDO | GND | TCK | 2V8 | TMS | GPS / ANT | WI-FI/BT / ANT | SIM/microSD / combo | GSM / ANT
